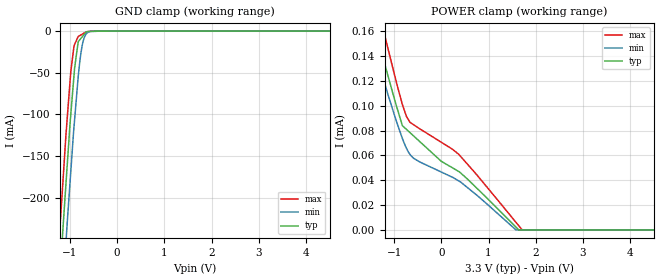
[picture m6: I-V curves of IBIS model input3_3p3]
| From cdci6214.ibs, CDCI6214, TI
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|   input3_3p3 Model
[Model]   input3_3p3
Model_type   Input
Vinl = 0.66
Vinh = 2.64
|   typ   min   max
C_comp   6.877E-13   6.696E-13   7.051E-13
|  Where Nom  PVT is Nominal Process, 3.3V,   32C
|   Fast PVT is Strong Process,  3.465V, -35C
|   Slow PVT is Weak Process,   3.135V,  110C
[Model spec]
|subparameter
Vinl   0.66   0.627   0.693
Vinh   2.64   2.508   2.772
[Voltage Range]   3.3   3.135   3.465
|Junction Temperature
[Temperature Range]   32   110   -35
[Power Clamp Reference]   3.3   3.135   3.465
[GND Clamp Reference]   0   0   0
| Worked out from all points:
|   GND clamp passes 1 mA (typ) near -0.65 V on its own axis
[GND Clamp]
|   Voltage   I(typ)   I(min)   I(max)
-3.3V     -2.319A    -2.382A    -2.268A
-1.236V   -318.5mA   -389.3mA   -258.7mA
-1.145V   -235.2mA   -308.4mA   -178.4mA
-1.086V   -186mA     -256.5mA   -126.9mA
-1.055V   -159.8mA   -229mA     -103.8mA
-981.4mV  -100.4mA   -169.1mA   -49.03mA
-900.4mV  -44.41mA   -106.4mA   -16.06mA
-824.2mV  -12.69mA   -54.78mA   -6.514mA
-768.1mV  -8.823mA   -27.15mA   -4.653mA
-714.6mV  -5.133mA   -11.11mA   -2.894mA
-651.9mV  -802.2uA   -3.263mA   -1.012mA
6.6V      0A         0A         0A
[POWER Clamp]
|   Voltage   I(typ)   I(min)   I(max)
-3.3V     444.8uA    396.4uA    509.5uA
-1.688V   203.7uA    180.5uA    235.7uA
-1.433V   167.2uA    147.8uA    194.3uA
-1.212V   135.5uA    119.6uA    159.2uA
-824.2mV  83.97uA    73.6uA     101uA
-738.8mV  81uA       65.87uA    91.48uA
-666.6mV  78.49uA    61.05uA    86.9uA
-474.1uV  55.3uA     46.67uA    70.63uA
357.9mV   47.34uA    39.76uA    61.29uA
1.583V    2.222uA    1.516nA    6.081uA
1.713V    0A         1.218nA    22.56nA
6.6V      0A         0A         0A
